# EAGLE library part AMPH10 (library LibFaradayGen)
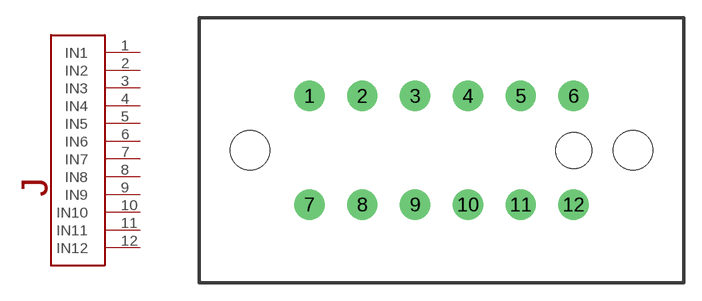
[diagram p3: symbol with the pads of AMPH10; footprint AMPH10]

Designator prefix J

## AMPH10  [AMPH10]
1  IN1  pas
2  IN2  pas
3  IN3  pas
4  IN4  pas
5  IN5  pas
6  IN6  pas
7  IN7  pas
8  IN8  pas
9  IN9  pas
10  IN10  pas
11  IN11  pas
12  IN12  pas

## Footprint AMPH10 (pad centres in mm)
drill 1.7: 1 -11.05,4.55; 2 -6.63,4.55; 3 -2.21,4.55; 4 2.21,4.55; 5 6.63,4.55; 6 11.05,4.55; 7 -11.05,-4.55; 8 -6.63,-4.55; 9 -2.21,-4.55; 10 2.21,-4.55; 11 6.63,-4.55; 12 11.05,-4.55
hole 3 at 11.05,0
hole 3.3 at 16.025,0
hole 3.3 at -16.025,0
